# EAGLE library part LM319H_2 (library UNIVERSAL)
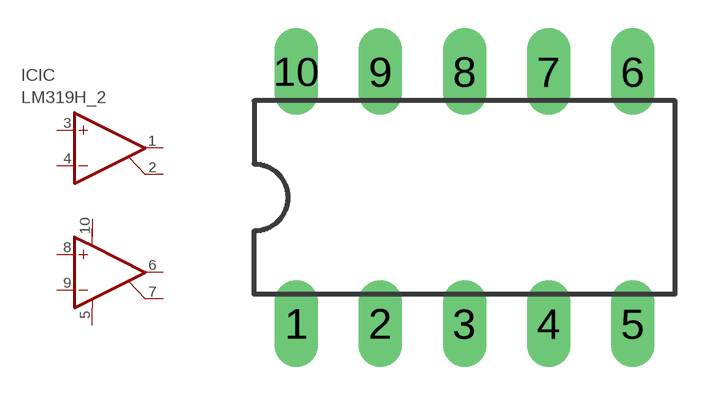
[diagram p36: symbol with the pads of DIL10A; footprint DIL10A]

Designator prefix IC; gates IC=KOMP_A G$2=KOMP_B

## LM319H_2  [DIL10A]
1  IC:OUT  out
2  IC:GNDA  pwr
3  IC:+INA  in
4  IC:-INB  in
5  G$2:V-  pwr
6  G$2:OUTB  out
7  G$2:GNDB  pwr
8  G$2:+INC  in
9  G$2:-IND  in
10  G$2:V+  pwr

## Footprint DIL10A (pad centres in mm)
drill 0.813 long: 1 0,0; 2 2.54,0; 3 5.08,0; 4 7.62,0; 5 10.16,0; 6 10.16,7.62; 7 7.62,7.62; 8 5.08,7.62; 9 2.54,7.62; 10 0,7.62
